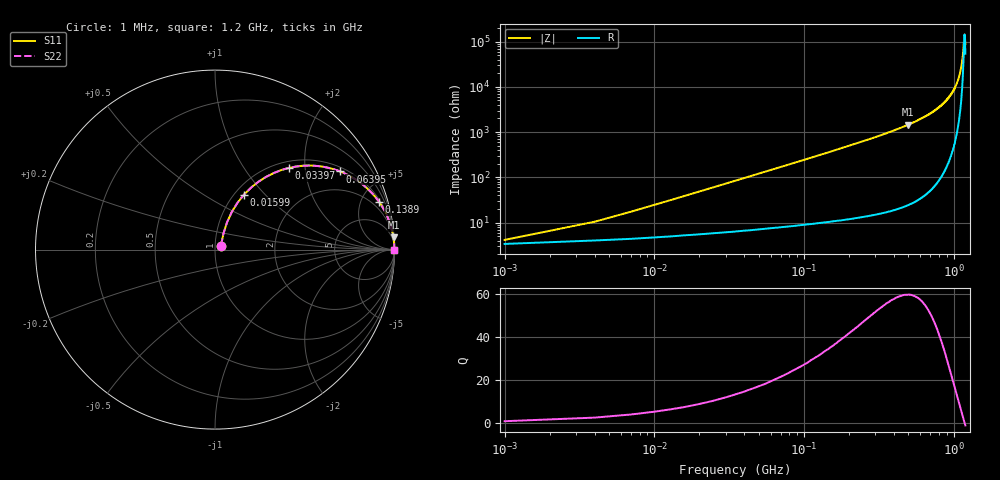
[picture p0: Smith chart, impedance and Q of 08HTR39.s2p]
! Coilcraft 0805HT-R39 Chip Inductor
! 6 August 2004
# MHZ S MA R 50
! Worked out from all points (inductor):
!   401 points, 1 MHz to 1.2 GHz, reference 50 ohm
!   read as one part in series: L = 384 nH near 6.995 MHz
!   highest Q = 59.8 at 498.6 MHz (marker M1), where L = 468 nH
!   self-resonance near 1.182 GHz
!   S11 on the Smith chart (normalised r, x): 1 MHz: 1.07, +0.05; 15.99 MHz: 1.10, +0.77; 33.97 MHz: 1.13, +1.64; 63.95 MHz: 1.15, +3.10; 138.9 MHz: 1.20, +6.80; 1.2 GHz: open
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1  0.04 34.0  0.967 -1.3  0.967 -1.3  0.04 34.0
9.992  0.229 66.0  0.931 -13.0  0.931 -13.0  0.229 66.0
15.987  0.347 62.2  0.892 -20.1  0.892 -20.1  0.347 62.2
24.98  0.497 54.8  0.821 -29.7  0.821 -29.7  0.497 54.8
33.972  0.613 47.9  0.745 -37.6  0.745 -37.6  0.613 47.9
48.96  0.743 38.7  0.627 -47.9  0.627 -47.9  0.743 38.7
63.948  0.822 32.0  0.53 -55.2  0.53 -55.2  0.822 32.0
93.923  0.903 23.3  0.396 -64.5  0.396 -64.5  0.903 23.3
138.885  0.952 16.3  0.28 -72.0  0.28 -72.0  0.952 16.3
201.833  0.976 11.2  0.195 -77.4  0.195 -77.4  0.976 11.2
402.665  0.994 5.2  0.091 -83.8  0.091 -83.8  0.994 5.2
498.585  0.997 3.9  0.068 -85.1  0.068 -85.1  0.997 3.9
600.5  0.998 2.9  0.051 -86.1  0.051 -86.1  0.998 2.9
801.332  0.999 1.6  0.028 -87.0  0.028 -87.0  0.999 1.6
930.225  0.999 1.0  0.017 -86.9  0.017 -86.9  0.999 1.0
1002.165  0.999 0.7  0.012 -86.2  0.012 -86.2  0.999 0.7
1071.107  0.999 0.4  0.007092 -84.3  0.007092 -84.3  0.999 0.4
1119.067  0.999 0.2  0.004045 -80.2  0.004045 -80.2  0.999 0.2
1149.042  0.999 0.1  0.002246 -72.2  0.002246 -72.2  0.999 0.1
1182.015  0.999 0.0  0.0007125 -13.1  0.0007125 -13.1  0.999 0.0
1188.01  0.999 -0.0  0.0007223 15.4  0.0007223 15.4  0.999 -0.0
1200  0.999 -0.1  0.001136 51.8  0.001136 51.8  0.999 -0.1
